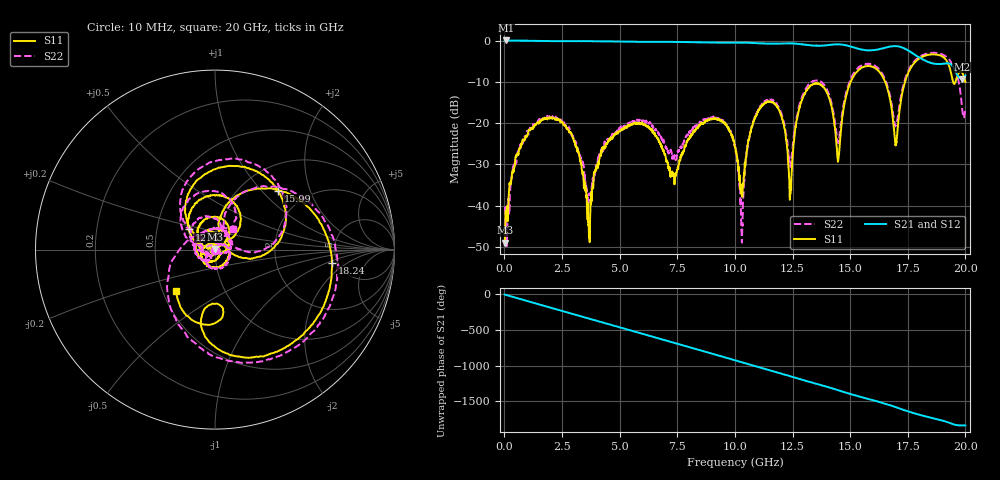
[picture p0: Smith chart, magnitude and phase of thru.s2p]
!Keysight Technologies,M9375A,MY57050901,A.13.90.07
!Date: Wednesday, January 06, 2021 09:17:45
!Correction: S11(C  2-Port  )
!S21(C  2-Port  )
!S12(C  2-Port  )
!S22(C  2-Port  )
!S2P File: Measurement: :
# Hz S  dB  R 50
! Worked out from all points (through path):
!   2000 points, 10 MHz to 20 GHz, reference 50 ohm
!   highest |S21| = 0.06 dB at 70 MHz (marker M1); lowest = -9.3 dB at 19.84 GHz (marker M2)
!   group delay of S21, straight-line fit = 260 ps
!   lowest |S11| = -49.0 dB at 30 MHz (marker M3), VSWR 1.01, Z = 49.8 + j0.303 ohm
!   |S11| at or under -10 dB: start of sweep to 15.02 GHz; 16.52 GHz to 17.38 GHz (856.2 MHz wide, 5.05 % of centre); 19.47039 GHz to 19.56474 GHz (94.35 MHz wide, 0.483 % of centre)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
!   |S22| runs from -49.8 to -2.9 dB; largest |S21 - S12| = 0.01
!   S11 on the Smith chart (normalised r, x): 10 MHz: 0.99, +0.00; 12.89 GHz: 0.73, +0.17; 15.99 GHz: 1.46, +1.24; 18.24 GHz: 4.49, -1.18; 20 GHz: 0.59, -0.30
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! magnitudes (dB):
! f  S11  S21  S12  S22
! 10 MHz  -46.5  0.0  0.0  -49.7
! 30 MHz  -49.0  0.0  0.1  -43.9
! 70 MHz  -43.5  0.1  0.1  -40.9
! 1.44 GHz  -19.8  -0.1  -0.1  -19.6
! 3.35 GHz  -30.8  -0.1  -0.1  -29.3
! 3.66 GHz  -44.5  -0.1  -0.1  -39.0
! 4.54 GHz  -24.1  -0.2  -0.2  -24.1
! 6.68 GHz  -23.8  -0.3  -0.3  -22.5
! 10.01 GHz  -25.7  -0.5  -0.5  -25.8
! 10.29 GHz  -36.6  -0.5  -0.5  -46.2
! 10.74 GHz  -20.7  -0.5  -0.5  -20.5
! 11.63 GHz  -14.9  -0.7  -0.7  -14.4
! 12.4 GHz  -36.8  -0.6  -0.6  -30.1
! 12.89 GHz  -14.7  -0.9  -0.8  -14.1
! 13.34 GHz  -10.7  -1.2  -1.1  -9.9
! 14.48 GHz  -29.1  -0.9  -0.9  -24.9
! 15.99 GHz  -6.4  -2.3  -2.3  -5.9
! 16.67 GHz  -12.6  -1.5  -1.5  -12.0
! 16.99 GHz  -25.2  -1.3  -1.3  -20.5
! 18.24 GHz  -3.7  -4.8  -4.8  -3.3
! 19.84 GHz  -7.6  -9.3  -9.3  -15.3
! 20 GHz  -10.0  -8.4  -8.4  -16.2
